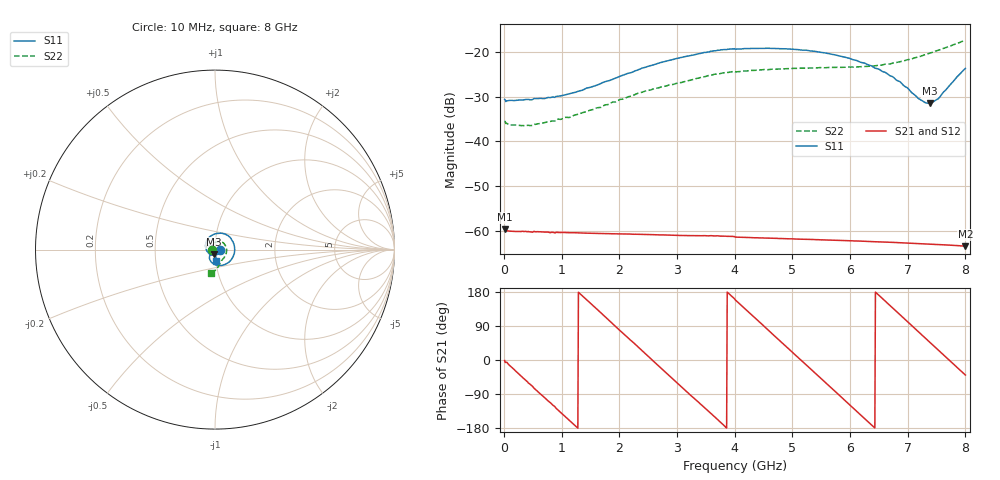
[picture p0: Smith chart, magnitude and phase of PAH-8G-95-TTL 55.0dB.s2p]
! MTS Systemtechnik GmbH
! S-Parameters
! Model: PAH-8G/95-TTL
! Attenuation Step: 55.0dB
! Rohde & Schwarz ZVB8 2Ports - Version 4.11 - 1145.1010k08 SN: 100119
! S2P File Measurements:
! S11 S21 S12 S22
# HZ  S  DB  R  50.00
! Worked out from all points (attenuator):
!   800 points, 10 MHz to 8 GHz, reference 50 ohm
!   highest |S21| = -59.69 dB at 10 MHz (marker M1); lowest = -63.5 dB at 8 GHz (marker M2)
!   lowest |S11| = -31.5 dB at 7.38 GHz (marker M3), VSWR 1.05, Z = 49.1 - j2.51 ohm
!   |S11| at or under -10 dB: start of sweep to end of sweep
!   |S22| runs from -36.5 to -17.4 dB; largest |S21 - S12| = 1.6e-05
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1e7  -30.60 -4.2  -59.69 -1.4  -59.60 -1.1  -35.56 -172.3
1.2e8  -30.82 -11.8  -60.13 -17.7  -60.14 -17.6  -36.35 174.6
4.7e8  -30.70 -45.6  -60.29 -66.6  -60.31 -66.3  -36.45 161.3
9e8  -29.97 -89.5  -60.38 -127.0  -60.39 -127.2  -35.17 149.5
1.35e9  -28.61 -135.7  -60.53 170.4  -60.54 170.4  -33.63 137.0
2.05e9  -25.25 163.1  -60.74 72.4  -60.75 72.5  -30.58 113.1
2.68e9  -22.50 117.5  -60.94 -15.6  -60.94 -15.3  -28.01 89.7
3.44e9  -20.21 69.1  -61.13 -120.6  -61.17 -121.0  -25.62 58.0
4.01e9  -19.36 33.0  -61.45 158.5  -61.45 158.5  -24.45 33.0
4.67e9  -19.18 -7.4  -61.72 66.5  -61.74 66.5  -23.85 5.1
5.34e9  -19.79 -48.4  -61.98 -26.8  -62.00 -26.8  -23.56 -22.1
5.73e9  -20.61 -72.0  -62.16 -81.1  -62.17 -81.3  -23.46 -36.1
6.11e9  -21.88 -95.0  -62.32 -134.7  -62.34 -134.6  -23.33 -47.9
6.36e9  -23.05 -109.1  -62.45 -169.6  -62.46 -169.7  -23.15 -54.4
6.67e9  -25.14 -123.9  -62.60 146.9  -62.62 146.9  -22.71 -61.7
6.87e9  -26.70 -130.3  -62.72 118.8  -62.73 118.8  -22.14 -66.6
7.2e9  -30.53 -124.6  -62.89 72.5  -62.91 72.5  -21.05 -74.6
7.31e9  -31.37 -114.7  -62.95 57.0  -62.97 57.0  -20.57 -77.4
7.38e9  -31.46 -107.3  -63.02 47.3  -63.03 47.2  -20.28 -79.1
7.54e9  -30.35 -91.7  -63.12 24.8  -63.12 24.8  -19.58 -83.9
7.86e9  -25.49 -83.1  -63.35 -20.1  -63.37 -20.1  -18.07 -94.7
8e9  -23.68 -86.0  -63.48 -39.7  -63.51 -39.6  -17.41 -100.1
